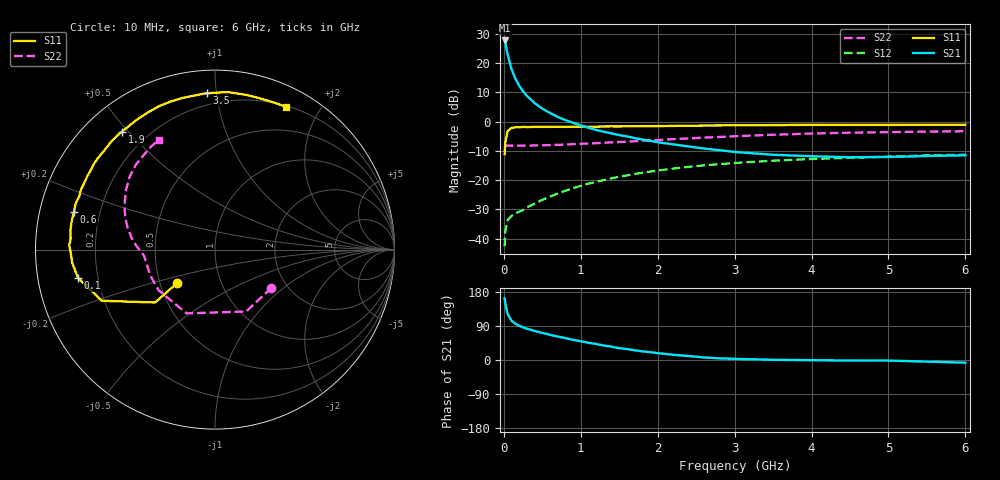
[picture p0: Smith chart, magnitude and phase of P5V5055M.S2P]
! SIEMENS Small Signal Semiconductors
! BFP183
! Si NPN RF Bipolar Junction Transistor in SOT143
! VCE = 0.5 V  IC = 55 mA
! Common Emitter S-Parameters:  March  1996
# GHz  S  MA  R  50
!  f  S11  S21  S12  S22
! GHz  MAG  ANG  MAG  ANG  MAG  ANG  MAG  ANG
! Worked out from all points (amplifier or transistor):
!   36 points, 10 MHz to 6 GHz, reference 50 ohm
!   highest |S21| = 27.8 dB at 10 MHz (marker M1)
!   |S21| within 3 dB of that: start of sweep to 35.79 MHz
!   unconditionally stable (mu >= 1): start of sweep to 32.44 MHz; 111.3 MHz to end of sweep
!   at 250 MHz: K = 1.59, MAG = 15.8 dB, |S12| = -30.2 dB
!   at 1.4 GHz: K = 2.14, MAG = 1.6 dB, |S12| = -19.4 dB
!   at 6 GHz: K = 1.41, MAG = -3.9 dB, |S12| = -11.3 dB
!   S11 on the Smith chart (normalised r, x): 10 MHz: 0.61, -0.25; 100 MHz: 0.13, -0.10; 600 MHz: 0.10, +0.13; 1.9 GHz: 0.11, +0.48; 3.5 GHz: 0.13, +0.94; 6 GHz: 0.21, +1.60
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0.01  0.2803 -138.6  24.49 162.8  0.0074 57.7  0.3798 -34.1
0.02  0.4449 -138.5  21.96 148.0  0.0136 52.5  0.386 -63.3
0.05  0.6925 -155.7  14.02 121.0  0.0209 38.6  0.3889 -114.0
0.1  0.7794 -168.4  7.913 103.6  0.0244 31.7  0.3871 -144.0
0.15  0.7991 -174.7  5.434 95.5  0.027 34.1  0.387 -155.7
0.2  0.8033 -178.3  4.101 90.2  0.0287 37.3  0.3876 -161.7
0.25  0.8126 178.3  3.311 86.0  0.0309 40.7  0.3878 -165.3
0.3  0.8068 175.8  2.761 82.6  0.0341 44.0  0.3883 -167.8
0.4  0.8129 172.2  2.078 76.6  0.0395 49.2  0.3914 -171.1
0.5  0.8142 168.6  1.665 71.5  0.0459 51.4  0.394 -173.1
0.6  0.8131 165.0  1.407 66.5  0.0522 53.6  0.3966 -174.8
0.7  0.8178 161.9  1.204 61.8  0.0589 55.1  0.4007 -176.0
0.8  0.8126 158.8  1.063 57.7  0.0657 55.7  0.4049 -176.9
1.1  0.821 149.7  0.786 45.4  0.0869 55.1  0.4227 179.9
1.5  0.827 139.4  0.589 31.2  0.1144 51.8  0.4476 175.5
1.9  0.8369 128.3  0.472 20.8  0.1396 46.8  0.4776 170.2
2.2  0.845 120.8  0.409 13.8  0.1574 42.7  0.5023 165.9
2.8  0.861 106.6  0.325 4.4  0.1874 34.0  0.5466 156.9
3.5  0.8727 93.1  0.271 0.5  0.2148 24.6  0.5965 146.3
4.5  0.8796 78.3  0.246 -1.4  0.2404 12.8  0.6477 132.6
5.5  0.8828 67.9  0.258 -4.3  0.2652 3.0  0.6755 122.0
6  0.8883 63.5  0.266 -7.1  0.2725 -2.0  0.686 117.3
